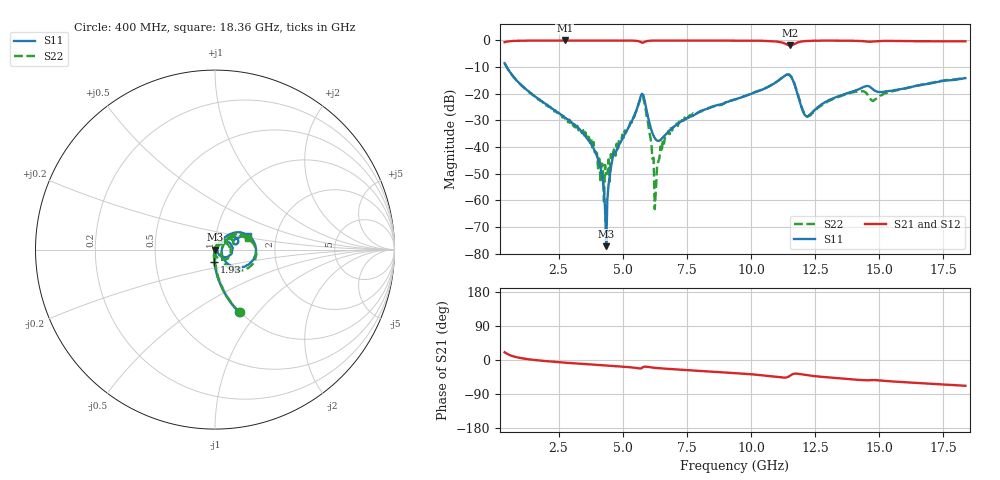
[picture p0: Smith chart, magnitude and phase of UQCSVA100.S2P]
!  Part Number  UQCSVA100  Mounting Orientation: Horizontal
!  Description: Ultra Low ESR Microwave capacitors
!  Application: Coupling, Bypass, Tuning, DC Block
!  Filters, Matching
# GHZ S DB R 50
! Freq  |S11|  S11 Ph  |S21|  S21 Ph  |S12|  S12 Ph  |S22|  S22 Ph
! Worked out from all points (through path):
!   400 points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, 400 MHz to 18.36 GHz, reference 50 ohm
!   highest |S21| = -0.02 dB at 2.74 GHz (marker M1); lowest = -1.9 dB at 11.52 GHz (marker M2)
!   group delay of S21, straight-line fit = 11.2 ps
!   lowest |S11| = -77.2 dB at 4.36 GHz (marker M3), VSWR 1.00, Z = 50 + j0.0074 ohm
!   |S11| at or under -10 dB: 483.5 MHz to end of sweep
!   |S22| runs from -63.3 to -8.5 dB; largest |S21 - S12| = 0.0032
!   S11 on the Smith chart (normalised r, x): 400 MHz: 0.98, -0.80; 1.93 GHz: 0.98, -0.13; 18.36 GHz: 1.42, +0.22
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0.4  -8.53 -69.1  -0.68 20.6  -0.69 20.6  -8.54 -68.6
1.93  -23.41 -93.0  -0.03 -2.4  -0.04 -2.4  -23.68 -92.4
2.74  -28.92 -99.9  -0.02 -7.0  -0.03 -6.9  -29.24 -88.2
3.415  -34.40 -105.3  -0.02 -10.2  -0.03 -10.2  -34.84 -95.4
4.09  -46.10 -108.9  -0.03 -13.2  -0.03 -13.2  -43.49 -81.8
4.135  -47.86 -109.0  -0.03 -13.5  -0.03 -13.4  -53.32 -36.4
4.18  -49.71 -106.0  -0.03 -13.7  -0.03 -13.6  -46.15 -96.3
4.27  -55.84 -107.2  -0.03 -14.1  -0.03 -14.0  -60.41 -103.5
4.315  -63.59 -100.0  -0.03 -14.3  -0.03 -14.2  -46.70 -22.1
4.36  -77.21 32.5  -0.03 -14.5  -0.03 -14.4  -50.24 56.4
4.405  -59.49 66.6  -0.03 -14.7  -0.03 -14.6  -49.85 -20.9
4.63  -42.91 67.7  -0.03 -15.7  -0.03 -15.6  -42.17 30.9
5.71  -20.82 24.2  -0.65 -22.1  -0.65 -22.0  -21.18 6.5
6.205  -35.81 -32.1  -0.07 -20.4  -0.06 -20.3  -44.05 -93.0
6.25  -36.68 -24.6  -0.06 -20.7  -0.06 -20.6  -63.33 48.9
6.385  -37.69 -1.2  -0.05 -21.5  -0.05 -21.4  -45.60 100.9
6.88  -33.33 40.9  -0.04 -23.9  -0.03 -23.8  -32.86 66.2
9.4  -22.11 51.4  -0.09 -34.5  -0.08 -34.4  -22.09 43.4
11.515  -13.11 -14.7  -1.91 -41.9  -1.90 -41.8  -12.94 -21.2
12.37  -27.18 21.6  -0.15 -41.8  -0.14 -41.7  -27.37 14.9
15.385  -18.98 24.5  -0.19 -56.0  -0.18 -56.0  -19.39 42.0
18.355  -14.16 22.1  -0.34 -68.1  -0.33 -68.1  -14.09 19.6
